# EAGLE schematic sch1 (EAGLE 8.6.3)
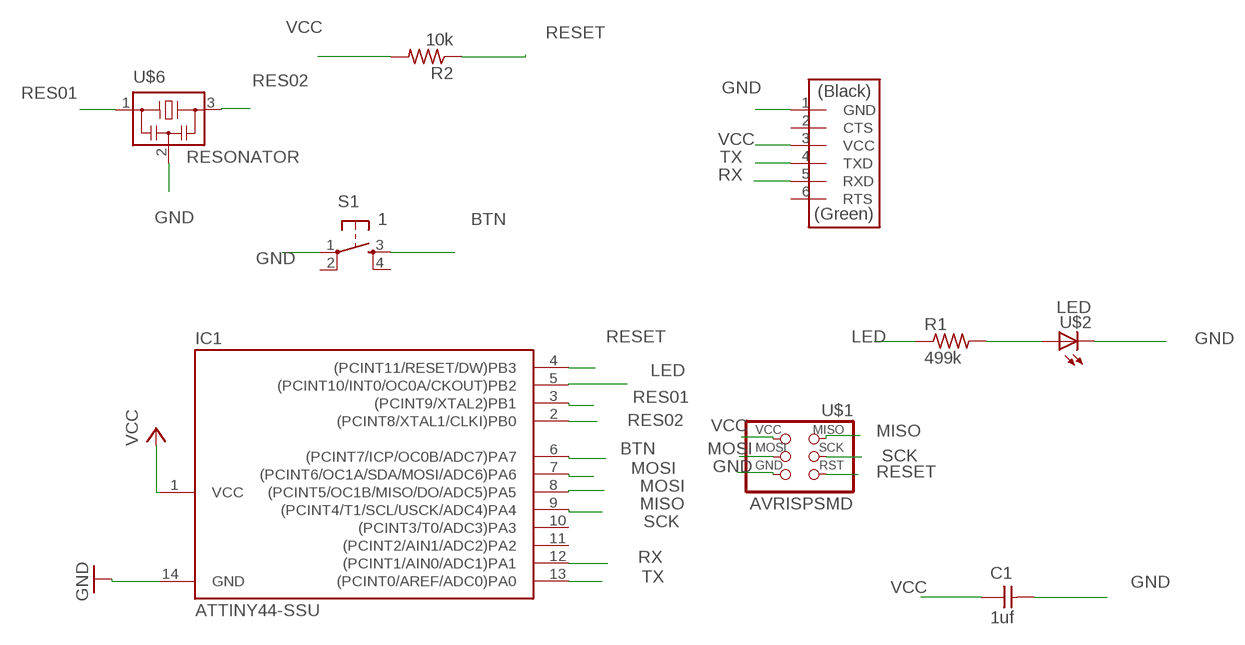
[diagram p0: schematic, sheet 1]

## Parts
C1  1uf  CAP-UNPOLARIZEDFAB  [C1206FAB]
IC1  ATTINY44-SSU  [SOIC14]
R1  499k  R-US_WSC2515  [WSC2515]
R2  10k  R-US_WSC2515  [WSC2515]
S1  1  6MM_SWITCH6MM_SWITCH  [6MM_SWITCH]
U$1  AVRISPSMD  [2X03SMD]
U$2  LED  [LED1206]
U$5  FTDI-SMD-HEADER  [1X06SMD]
U$6  RESONATOR  [EFOBM]

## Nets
BTN: IC1.6((PCINT7/ICP/OC0B/ADC7)PA7) S1.3(S)
GND: C1.2 IC1.14(GND) S1.1(P) U$1.6(GND) U$2.2(C) U$5.1(GND) U$6.2
LED: IC1.5((PCINT10/INT0/OC0A/CKOUT)PB2) R1.1
MISO: IC1.8((PCINT5/OC1B/MISO/DO/ADC5)PA5) U$1.1(MISO)
MOSI: IC1.7((PCINT6/OC1A/SDA/MOSI/ADC6)PA6) U$1.4(MOSI)
N$2: R1.2 U$2.1(A)
RES01: IC1.3((PCINT9/XTAL2)PB1) U$6.1
RES02: IC1.2((PCINT8/XTAL1/CLKI)PB0) U$6.3
RESET: IC1.4((PCINT11/RESET/DW)PB3) R2.1 U$1.5(RST)
RX: IC1.12((PCINT1/AIN0/ADC1)PA1) U$5.5(RXD)
SCK: IC1.9((PCINT4/T1/SCL/USCK/ADC4)PA4) U$1.3(SCK)
TX: IC1.13((PCINT0/AREF/ADC0)PA0) U$5.4(TXD)
VCC: C1.1 IC1.1(VCC) R2.2 U$1.2(VCC) U$5.3(VCC)
Unconnected: IC1.10((PCINT3/T0/ADC3)PA3) IC1.11((PCINT2/AIN1/ADC2)PA2) S1.2(P1) S1.4(S1) U$5.2(CTS) U$5.6(RTS)

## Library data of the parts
C1 = fab:CAP-UNPOLARIZED
IC1 = fab:ATTINY44
R1 R2 = resistor:R-US_: RESISTOR, American symbol
S1 = fab:6MM_SWITCH: OMRON SWITCH
U$1 = fab:AVRISP
U$2 = fab:LED: LED
U$5 = fab:FTDI-SMD-HEADER
U$6 = fab:RESONATOR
